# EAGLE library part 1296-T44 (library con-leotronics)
1.27mm SINGLE ROW FEMALE SOCKET Source: http://www.leotronics.co.uk/Conexcon/Data%20Sheets/sec.%20A/1296ing.pdf
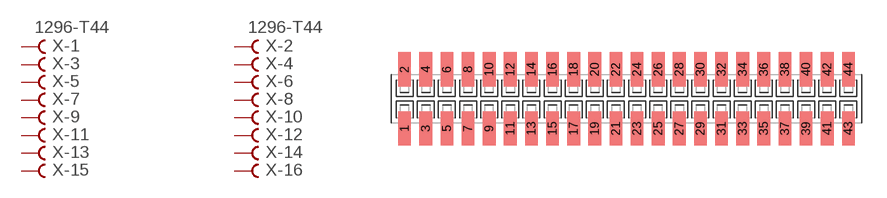
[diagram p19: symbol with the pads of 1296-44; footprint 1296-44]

Designator prefix X; gates -1=FVAL -2=FVAL -3=F -4=F -5=F -6=F -7=F -8=F -9=F -10=F -11=F -12=F -13=F -14=F -15=F -16=F -17=F -18=F -19=F -20=F -21=F -22=F -23=F -24=F -25=F -26=F -27=F -28=F -29=F -30=F -31=F -32=F -33=F -34=F -35=F -36=F -37=F -38=F -39=F -40=F -41=F -42=F -43=F -44=F

## 1296-T44 (OC_FARNELL: unknown; OC_NEWARK: unknown)  [1296-44]
1  -1:B  pas
2  -2:B  pas
3  -3:B  pas
4  -4:B  pas
5  -5:B  pas
6  -6:B  pas
7  -7:B  pas
8  -8:B  pas
9  -9:B  pas
10  -10:B  pas
11  -11:B  pas
12  -12:B  pas
13  -13:B  pas
14  -14:B  pas
15  -15:B  pas
16  -16:B  pas
17  -17:B  pas
18  -18:B  pas
19  -19:B  pas
20  -20:B  pas
21  -21:B  pas
22  -22:B  pas
23  -23:B  pas
24  -24:B  pas
25  -25:B  pas
26  -26:B  pas
27  -27:B  pas
28  -28:B  pas
29  -29:B  pas
30  -30:B  pas
31  -31:B  pas
32  -32:B  pas
33  -33:B  pas
34  -34:B  pas
35  -35:B  pas
36  -36:B  pas
37  -37:B  pas
38  -38:B  pas
39  -39:B  pas
40  -40:B  pas
41  -41:B  pas
42  -42:B  pas
43  -43:B  pas
44  -44:B  pas

## Footprint 1296-44 (pad centres in mm)
1.27mm SINGLE ROW FEMALE SOCKET Source: http://www.leotronics.co.uk/Conexcon/Data%20Sheets/sec.%20A/1296ing.pdf
smd 0.76 x 2.05: 1 -13.335,-1.78; 2 -13.335,1.78; 3 -12.065,-1.78; 4 -12.065,1.78; 5 -10.795,-1.78; 6 -10.795,1.78; 7 -9.525,-1.78; 8 -9.525,1.78; 9 -8.255,-1.78; 10 -8.255,1.78; 11 -6.985,-1.78; 12 -6.985,1.78; 13 -5.715,-1.78; 14 -5.715,1.78; 15 -4.445,-1.78; 16 -4.445,1.78; 17 -3.175,-1.78; 18 -3.175,1.78; 19 -1.905,-1.78; 20 -1.905,1.78; 21 -0.635,-1.78; 22 -0.635,1.78; 23 0.635,-1.78; 24 0.635,1.78; 25 1.905,-1.78; 26 1.905,1.78; 27 3.175,-1.78; 28 3.175,1.78; 29 4.445,-1.78; 30 4.445,1.78; 31 5.715,-1.78; 32 5.715,1.78; 33 6.985,-1.78; 34 6.985,1.78; 35 8.255,-1.78; 36 8.255,1.78; 37 9.525,-1.78; 38 9.525,1.78; 39 10.795,-1.78; 40 10.795,1.78; 41 12.065,-1.78; 42 12.065,1.78; 43 13.335,-1.78; 44 13.335,1.78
